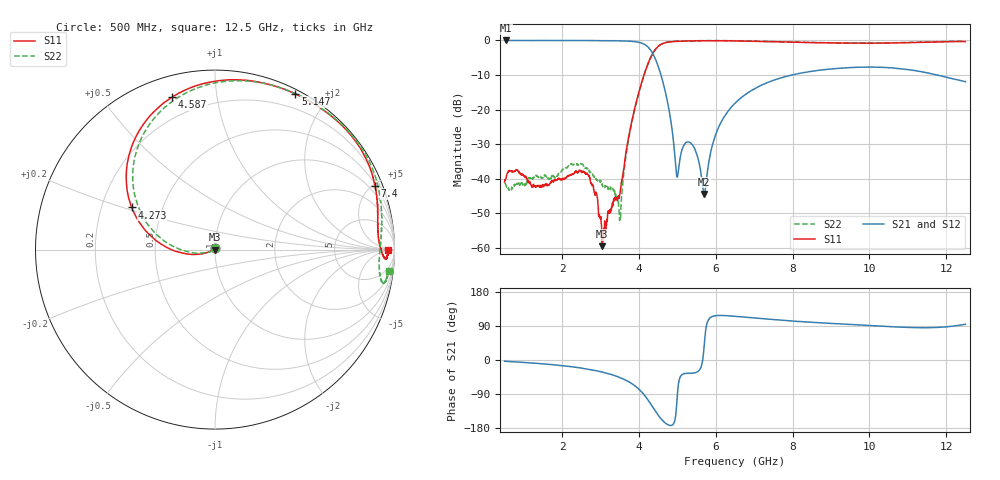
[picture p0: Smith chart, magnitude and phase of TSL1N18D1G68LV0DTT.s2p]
! TSL1N18D1G68LV0DTT  S-PARAMETER MODEL  ( General Type )
! Model Generated by TAIYO YUDEN Corporation (https://www.yuden.co.jp/en/)
! Version 1.0
! TAIYO YUDEN Control No. PG20171206-Z01
! Copyright(c) 2017 TAIYO YUDEN CO.,LTD. All Rights Reserved.
! Products Name : Multilayer Ceramic Devices
! Characteristics :
!  Passband freq : 617-2690MHz ( At Passband , Insertion Loss : 0.2dB , VSWR 1.5 ),
!  Attenuation : 25dB min at 5150-5950MHz , Impedance : 50 Ohm ,
!  Case Size : 1.6 x 0.8 / 0.063 x 0.031 [mm/inch] , Thickness : 0.65 / 0.026 [mm/inch]
!  (Conditions: Temperature = 25 degC , DC Bias Current/Voltage = 0A / 0V)
! External Node Assignments :
!  1  o---|-------|---o  2
!  |  LPF  |
! GND o---|-------|---o GND
! Frequency Range : 500MHz  -  12.5GHz  [ 1801 STEP ]
# MHZ S RI R 50
! Freq[MHz].  S11 Real  S11 Imag  S21 Real  S21 Imag  S12 Real  S12 Imag  S22 Real  S22 Imag
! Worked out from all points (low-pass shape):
!   1801 points, 500 MHz to 12.5 GHz, reference 50 ohm
!   highest |S21| = -0.01 dB at 540 MHz (marker M1); lowest = -44.4 dB at 5.7 GHz (marker M2)
!   |S21| within 3 dB of the highest: start of sweep to 4.315 GHz
!   lowest |S11| = -59.5 dB at 3.04 GHz (marker M3), VSWR 1.00, Z = 49.9 - j0.0578 ohm
!   |S11| at or under -10 dB: start of sweep to 4.13 GHz
!   |S22| runs from -52.0 to -0.1 dB; largest |S21 - S12| = 0.0026
!   S11 on the Smith chart (normalised r, x): 500 MHz: 1.00, +0.02; 4.273 GHz: 0.33, +0.21; 4.587 GHz: 0.10, +0.75; 5.147 GHz: 0.04, +1.64; 7.4 GHz: 0.56, +5.15; 12.5 GHz: 53, -2
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500  0.00171 0.00883  0.9959 -0.057  0.9965 -0.0577  0.00147 0.00849
540  0.00136 0.0102  0.9968 -0.0614  0.9974 -0.0614  0.00179 0.00767
1440  0.00713 0.0026  0.9828 -0.1679  0.9838 -0.1677  0.0107 -0.000256
2500  -0.0018 -0.0125  0.9275 -0.3623  0.9279 -0.3623  0.00468 -0.0158
2853.333  -0.00305 -0.00532  0.8808 -0.4599  0.8815 -0.4603  0.00409 -0.00909
3040  -0.000892 -0.000579  0.8439 -0.5222  0.844 -0.5222  0.00655 -0.00517
3506.667  -0.00576 0.00213  0.6782 -0.7135  0.678 -0.7138  0.00062 -0.00257
3806.667  -0.062 -0.0214  0.4559 -0.857  0.4559 -0.8575  -0.0599 -0.0177
4273.333  -0.464 0.2346  -0.2752 -0.7077  -0.2749 -0.7086  -0.4406 0.2779
4500  -0.3784 0.726  -0.349 -0.2374  -0.3499 -0.2385  -0.3138 0.7594
4586.667  -0.2376 0.8507  -0.2722 -0.1173  -0.2721 -0.1173  -0.1647 0.871
4800  0.1073 0.946  -0.086 -0.0111  -0.0857 -0.011  0.1833 0.9386
4980  0.3138 0.9172  -0.00529 -0.00973  -0.00528 -0.00964  0.3841 0.8953
5146.667  0.4483 0.8673  0.0231 -0.0173  0.023 -0.0175  0.511 0.8374
5433.333  0.6011 0.7791  0.0234 -0.0159  0.0235 -0.016  0.6544 0.7417
5700  0.6934 0.7046  0.00461 0.00392  0.00454 0.00386  0.7399 0.6621
6000  0.7637 0.6291  -0.0201 0.0395  -0.0202 0.0396  0.8043 0.583
6500  0.8348 0.5201  -0.0531 0.1121  -0.0528 0.1125  0.8697 0.4681
7400  0.892 0.3557  -0.0764 0.2407  -0.0759 0.2415  0.9202 0.2877
8500  0.906 0.2078  -0.0583 0.3531  -0.0585 0.3527  0.9273 0.1116
10500  0.9172 0.0315  0.0123 0.4029  0.0112 0.4033  0.9154 -0.1107
12500  0.9633 -0.00132  -0.0192 0.2529  -0.019 0.2525  0.9668 -0.1168
